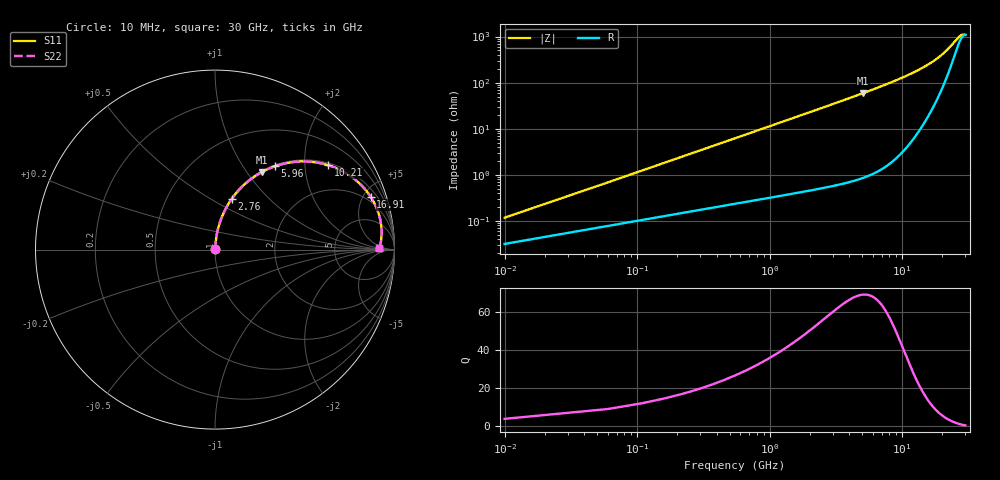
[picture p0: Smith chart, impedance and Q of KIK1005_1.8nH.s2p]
!version-3
!date-01.2023
!Series
# MHz S RI R 50
!Freq ReS11 ImS11 ReS21 ImS21 ReS12 ImS12 ReS22 ImS22
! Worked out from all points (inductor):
!   601 points, 10 MHz to 30 GHz, reference 50 ohm
!   read as one part in series: L = 1.8 nH near 160 MHz
!   highest Q = 69.1 at 5.06 GHz (marker M1), where L = 1.86 nH
!   S11 on the Smith chart (normalised r, x): 10 MHz: 1.00, +0.00; 2.76 GHz: 1.01, +0.63; 5.96 GHz: 1.02, +1.41; 10.21 GHz: 1.07, +2.63; 16.91 GHz: 1.55, +5.64; 30 GHz: 23, +2
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10  0.000317 0.00113  0.9997 -0.00113  0.9997 -0.00113  0.000317 0.00113
110  0.0012 0.0124  0.9988 -0.0124  0.9988 -0.0124  0.0012 0.0124
210  0.00201 0.0237  0.998 -0.0237  0.998 -0.0237  0.00201 0.0237
260  0.00247 0.0293  0.9975 -0.0293  0.9975 -0.0293  0.00247 0.0293
410  0.00416 0.0461  0.9958 -0.0461  0.9958 -0.0461  0.00416 0.0461
610  0.00717 0.0684  0.9928 -0.0684  0.9928 -0.0684  0.00717 0.0684
960  0.0147 0.1068  0.9853 -0.1068  0.9853 -0.1068  0.0147 0.1068
1410  0.0284 0.1547  0.9716 -0.1547  0.9716 -0.1547  0.0284 0.1547
2010  0.0535 0.2152  0.9465 -0.2152  0.9465 -0.2152  0.0535 0.2152
2760  0.0943 0.2837  0.9057 -0.2837  0.9057 -0.2837  0.0943 0.2837
5010  0.2573 0.43  0.7427 -0.43  0.7427 -0.43  0.2573 0.43
5060  0.2613 0.4322  0.7387 -0.4322  0.7387 -0.4322  0.2613 0.4322
5960  0.3334 0.4641  0.6666 -0.4641  0.6666 -0.4641  0.3334 0.4641
7810  0.4756 0.4909  0.5244 -0.4909  0.5244 -0.4909  0.4756 0.4909
10010  0.6191 0.4738  0.3809 -0.4738  0.3809 -0.4738  0.6191 0.4738
10210  0.6304 0.4704  0.3696 -0.4704  0.3696 -0.4704  0.6304 0.4704
15010  0.8244 0.3493  0.1756 -0.3493  0.1756 -0.3493  0.8244 0.3493
16910  0.8671 0.2946  0.1329 -0.2946  0.1329 -0.2946  0.8671 0.2946
20010  0.9087 0.2098  0.0913 -0.2098  0.0913 -0.2098  0.9087 0.2098
25010  0.9284 0.0945  0.0716 -0.0945  0.0716 -0.0945  0.9284 0.0945
27760  0.9243 0.0433  0.0757 -0.0433  0.0757 -0.0433  0.9243 0.0433
30000  0.9163 0.00746  0.0837 -0.00746  0.0837 -0.00746  0.9163 0.00746
